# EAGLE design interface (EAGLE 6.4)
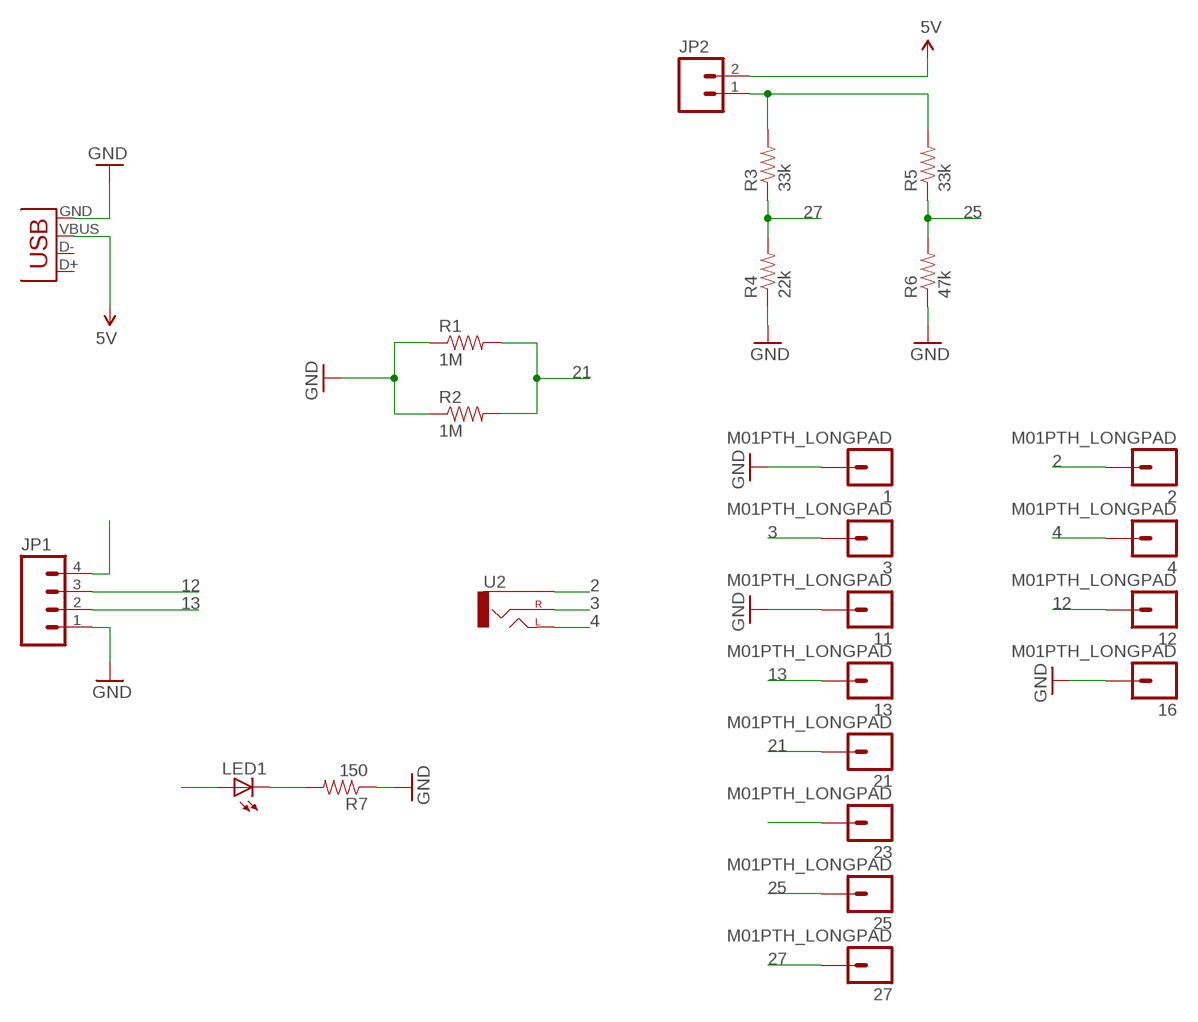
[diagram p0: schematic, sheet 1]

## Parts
1  M01PTH_LONGPAD  [1X01_LONGPAD]
2  M01PTH_LONGPAD  [1X01_LONGPAD]
3  M01PTH_LONGPAD  [1X01_LONGPAD]
4  M01PTH_LONGPAD  [1X01_LONGPAD]
11  M01PTH_LONGPAD  [1X01_LONGPAD]
12  M01PTH_LONGPAD  [1X01_LONGPAD]
13  M01PTH_LONGPAD  [1X01_LONGPAD]
16  M01PTH_LONGPAD  [1X01_LONGPAD]
21  M01PTH_LONGPAD  [1X01_LONGPAD]
23  M01PTH_LONGPAD  [1X01_LONGPAD]
25  M01PTH_LONGPAD  [1X01_LONGPAD]
27  M01PTH_LONGPAD  [1X01_LONGPAD]
JP1  M04PTH  [1X04]
JP2  M02PTH3  [1X02_LONGPADS]
LED1  LED5MM  [LED5MM]
R1  1M  RESISTORPTH-1/4W  [AXIAL-0.4]
R2  1M  RESISTORPTH-1/4W  [AXIAL-0.4]
R3  33k  RESISTORPTH-1/4W  [AXIAL-0.4]
R4  22k  RESISTORPTH-1/4W  [AXIAL-0.4]
R5  33k  RESISTORPTH-1/4W  [AXIAL-0.4]
R6  47k  RESISTORPTH-1/4W  [AXIAL-0.4]
R7  150  RESISTORPTH-1/4W  [AXIAL-0.4]
U2  AUDIO-JACKPTH  [AUDIO-JACK]
X1  USB-SMD-NS  [USB-MINIB-NOSTOP]

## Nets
2: 2.1 U2.SLEEVE
3: 3.1 U2.RING(RIGHT)
4: 4.1 U2.TIP(LEFT)
5V: JP2.2 X1.VBUS
12: 12.1 JP1.3
13: 13.1 JP1.2
21: 21.1 R1.P$2 R2.P$2
25: 25.1 R5.P$1 R6.P$2
27: 27.1 R3.P$1 R4.P$2
GND: 1.1 11.1 16.1 JP1.1 R1.P$1 R2.P$1 R4.P$1 R6.P$1 R7.P$1 X1.GND
N$1: LED1.K(C) R7.P$2
P_IN: 23.1 JP1.4 JP2.1 LED1.A R3.P$2 R5.P$2
Unconnected: X1.D+ X1.D-

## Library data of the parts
1-4 11-13 16 21 23 25 27 = SparkFun-Connectors:M01: Header 1
JP1 = SparkFun-Connectors:M04: Header 4 Standard 4-pin 0.1" header. Use with straight break away headers (SKU : PRT-00116), right angle break away headers (PRT-00553), swiss pins (PRT-00743), machine pins (PRT-00117), and female headers (PRT-00115). Molex polarized connector foot print use with SKU : PRT-08231 with associated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
JP2 = SparkFun-Connectors:M02: Header 2
LED1 = SparkFun-LED:LED: LEDs
R1-R7 = SparkFun-Passives:RESISTOR: Resistor
U2 = SparkFun-Connectors:AUDIO-JACK: 3.5mm Audio Jack Simple 3.5mm common PCB mount audio jack. SKU: PRT-08032
X1 = SparkFun-Connectors:USB: USB Connectors USB-B-PTH is fully proven SKU : PRT-00139 USB-miniB is fully proven SKU : PRT-00587 USB-A-PCB is untested. USB-A-H is throughly reviewed, but untested. Spark Fun Electronics SKU : PRT-00437 USB-B-SMT is throughly reviewed, but untested. Needs silkscreen touching up. USB-A-S has not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

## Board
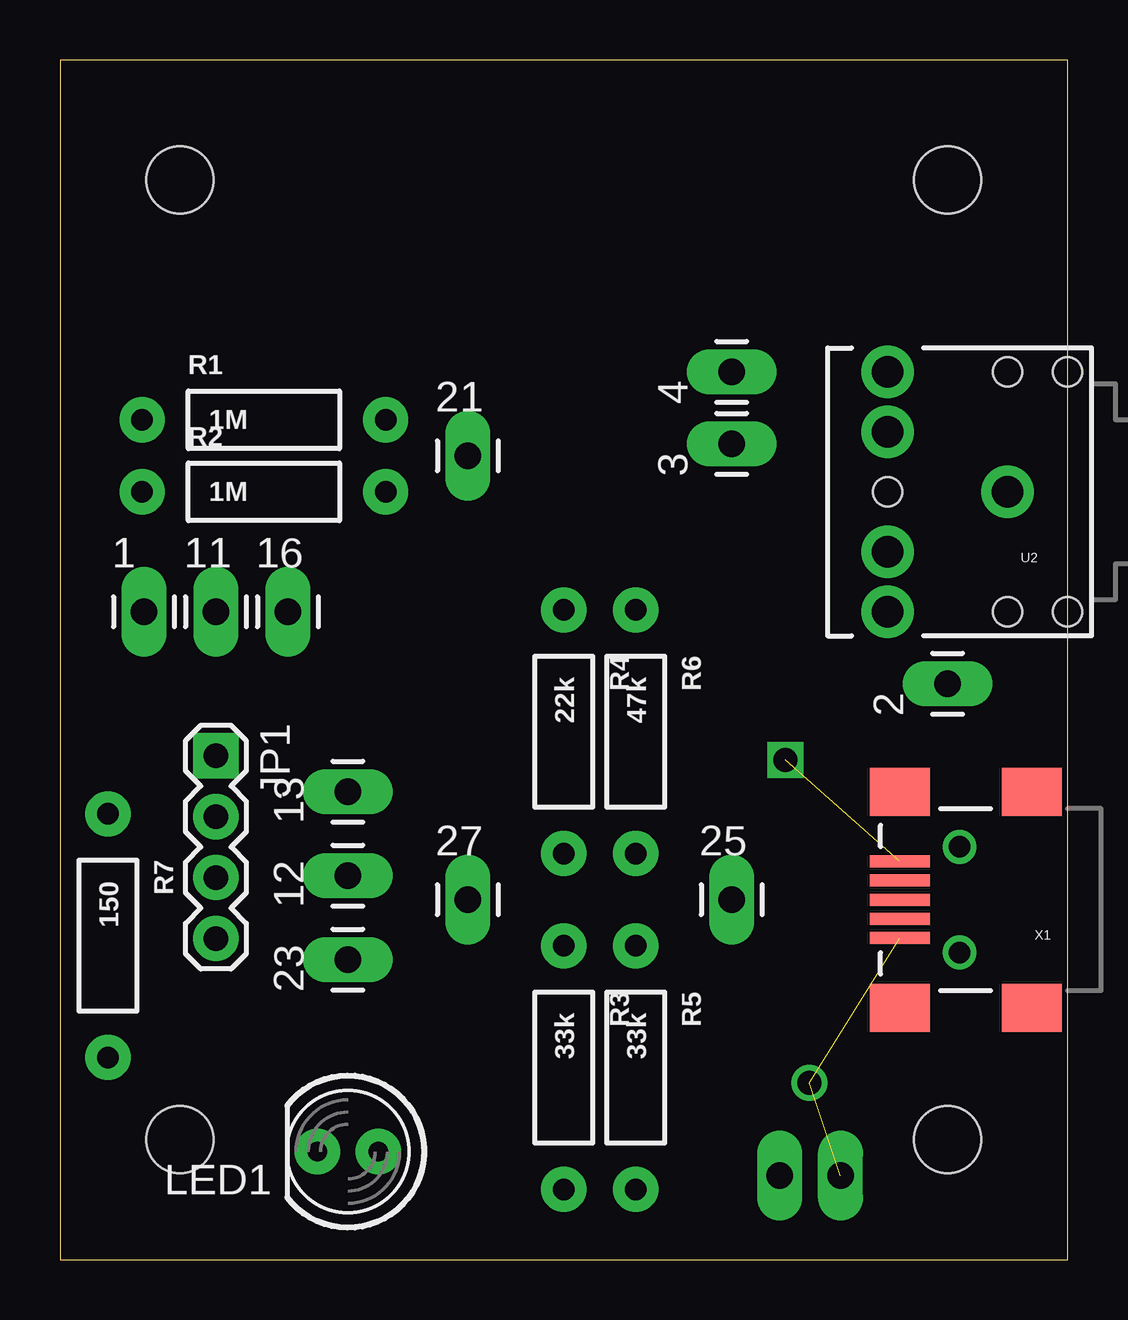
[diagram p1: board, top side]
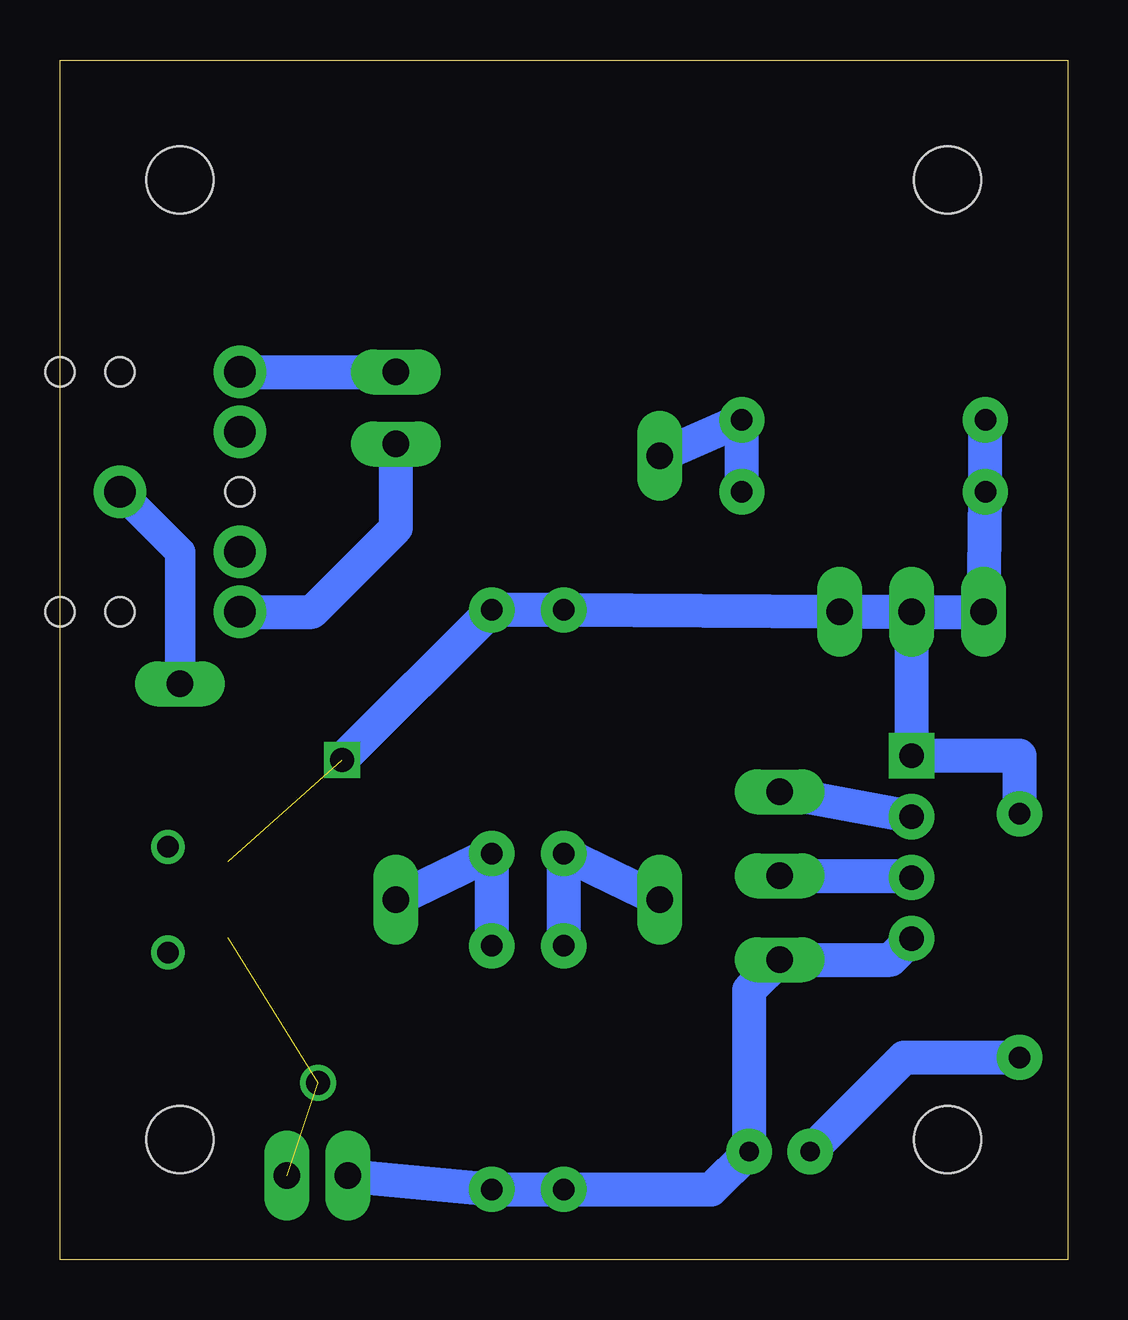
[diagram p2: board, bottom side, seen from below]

Size 42 x 50 mm. Coordinates in mm from the lower left corner, seen from the top.
Outline: 0,0 42,0 42,50 0,50 0,0
Copper layers (1*16): Top 0.035mm / dielectric 1.5mm / Bottom 0.035mm
Design rules "default": minimum track width 10mil, minimum drill 24mil, track to track 8mil, track to pad 8mil, pad to pad 8mil, via to via 8mil, smd to smd 8mil, copper to edge 40mil, drill to drill 8mil, minimum pad ring 10mil, minimum via ring 8mil, stop-mask expansion 4mil, vias tented up to drill 0mil, thermal gap 10mil
Holes 2.8 mm at 5,5 5,45 37,5 37,45

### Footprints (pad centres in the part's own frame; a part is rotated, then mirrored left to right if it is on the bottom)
1X01_LONGPAD = drill 1.118 pad 1.88 long: 1 0,0
1X04 = drill 1.016 pad 1.88 square: 1 0,0 | drill 1.016 pad 1.88: 2 2.54,0; 3 5.08,0; 4 7.62,0
1X02_LONGPADS = drill 1.118 pad 1.88 long: 1 0,0; 2 2.54,0
LED5MM = drill 0.813 pad 1.88: A -1.27,0; K 1.27,0
AXIAL-0.4 = drill 0.9 pad 1.88: P$1 -5.08,0; P$2 5.08,0
AUDIO-JACK = drill 1.3 pad 2.184: RING 5,5; RSH 5,2.5; SLEEVE 0,0; TIP 5,-5; TSH 5,-2.5 | hole 1.2: 0,5; -2.5,5; -2.5,-5; 0,-5; 5,0
USB-MINIB-NOSTOP = smd 2.5 x 0.5: D+ 2.5,0; D- 2.5,0.8; GND 2.5,-1.6; ID 2.5,-0.8; VBUS 2.5,1.6 | smd 2.5 x 2: G1 -3,-4.5; G2 -3,4.5; G3 2.5,4.5; G4 2.5,-4.5 | drill 0.9 pad 0.8: H1 0,2.2 | drill 0.9 pad 0.787: H2 0,-2.2

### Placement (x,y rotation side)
1  3.5,27 0 top
2  37,24 90 top
3  28,34 90 top
4  28,37 90 top
11  6.5,27 0 top
12  12,16 90 top
13  12,19.5 90 top
16  9.5,27 0 top
21  17,33.5 0 top
23  12,12.5 90 top
25  28,15 0 top
27  17,15 0 top
JP1  6.5,21 270 top
JP2  30,3.5 0 top
LED1  12,4.5 180 top
R1  8.5,35 0 top
R2  8.5,32 0 top
R3  21,8 270 top
R4  21,22 270 top
R5  24,8 270 top
R6  24,22 270 top
R7  2,13.5 270 top
U2  39.5,32 180 top
X1  37.5,15 180 top

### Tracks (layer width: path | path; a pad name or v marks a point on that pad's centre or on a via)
2
  Bottom 1.27: U2.SLEEVE 37,29.5 2.1
3
  Bottom 1.422: U2.RING 31.5,27 28,30.5 3.1
4
  Bottom 1.422: U2.TIP 4.1
5V  (via drill 1 pad 0.25)  (2 unrouted)
  other vias: 31.24,7.37
12
  Bottom 1.422: 12.1 6.58,16 JP1.3
13
  Bottom 1.422: 13.1 JP1.2
21
  Bottom 1.422: R2.P$2 R1.P$2 21.1
25
  Bottom 1.422: R5.P$1 R6.P$2 25.1
27
  Bottom 1.422: R3.P$1 R4.P$2 27.1
GND  (via drill 1)  (1 unrouted)
  Bottom 1.422: R7.P$1 2,21 JP1.1 11.1 | 11.1 1.1 R2.P$1 R1.P$1 | 11.1 16.1 R4.P$1 R6.P$1 v30.24,20.84 v30.24,20.83
N$1
  Bottom 1.422: LED1.K 6.81,8.42 R7.P$2
P_IN
  Bottom 1.422: JP2.1 R5.P$2 R3.P$2 14.85,2.92 LED1.A 13.27,11.23 23.1 7.38,12.5 JP1.4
